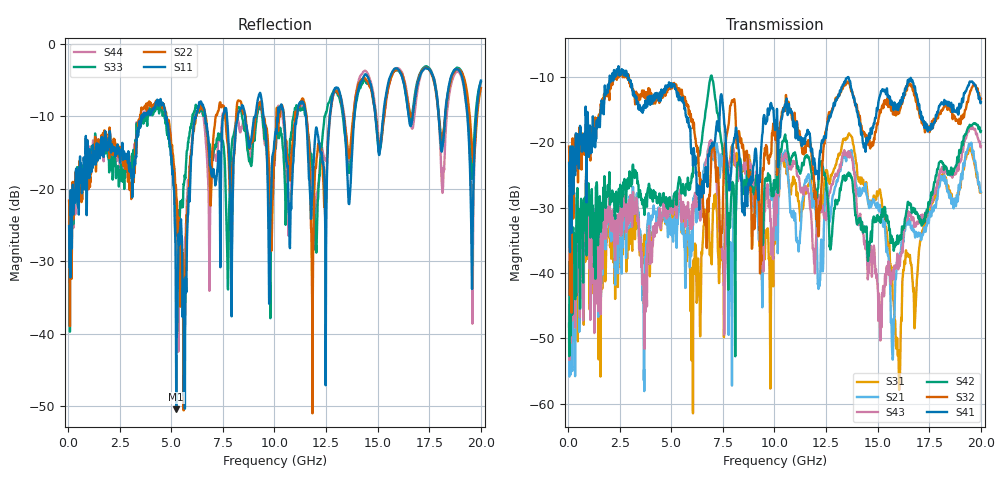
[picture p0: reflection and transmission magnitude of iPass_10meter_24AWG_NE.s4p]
! FILE: D:\iPass\iPassCables1205\10meter\iPass_10meter_24AWG_NE.s4p
# MHz S MA R 50.00
! FREQ  S11  S12  S13  S14
!  S21  S22  S23  S24
!  S31  S32  S33  S34
!  S41  S42  S43  S44
!  MAG  ANG  MAG  ANG  MAG  ANG  MAG  ANG
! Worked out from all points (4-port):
!   1996 points, 50 MHz to 20 GHz, reference 50 ohm
!   strongest paths, dB at 50 MHz, 5.04 GHz, 10.03 GHz, 15.02 GHz, 20 GHz:
!     S41: -23.2, -11.5, -18.1, -14.3, -13.9
!     S32: -20.7, -11.8, -19.2, -16.9, -13.3
!     S42: -47.7, -29.6, -26.0, -31.2, -18.3
!     S43: -46.7, -30.5, -28.1, -43.5, -20.6
!     S21: -50.3, -34.4, -32.7, -29.9, -27.6
!     S31: -48.0, -33.2, -35.5, -27.9, -27.7
!   lowest |S11| = -50.4 dB at 5.24 GHz (marker M1), VSWR 1.01, Z = 49.7 - j0.0666 ohm
!   |S11| at or under -10 dB: start of sweep to 3.553 GHz; 4.727 GHz to 6.191 GHz (1.464 GHz wide, 26.8 % of centre); 11.52 GHz to 12.68 GHz (1.155 GHz wide, 9.54 % of centre)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
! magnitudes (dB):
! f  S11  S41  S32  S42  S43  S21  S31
! 50 MHz  -25.1  -23.2  -20.7  -47.7  -46.7  -50.3  -48.0
! 4.51 GHz  -8.2  -12.1  -13.3  -28.8  -32.1  -31.4  -33.2
! 5.24 GHz  -50.4  -12.1  -11.2  -28.8  -29.1  -33.0  -30.9
! 6.41 GHz  -8.2  -28.1  -26.2  -21.2  -31.6  -30.2  -47.1
! 13.66 GHz  -20.8  -10.6  -11.4  -24.8  -21.5  -21.5  -18.9
! 16.01 GHz  -3.5  -14.5  -15.2  -35.2  -38.9  -38.2  -52.7
! 20 GHz  -5.0  -13.9  -13.3  -18.3  -20.6  -27.6  -27.7
